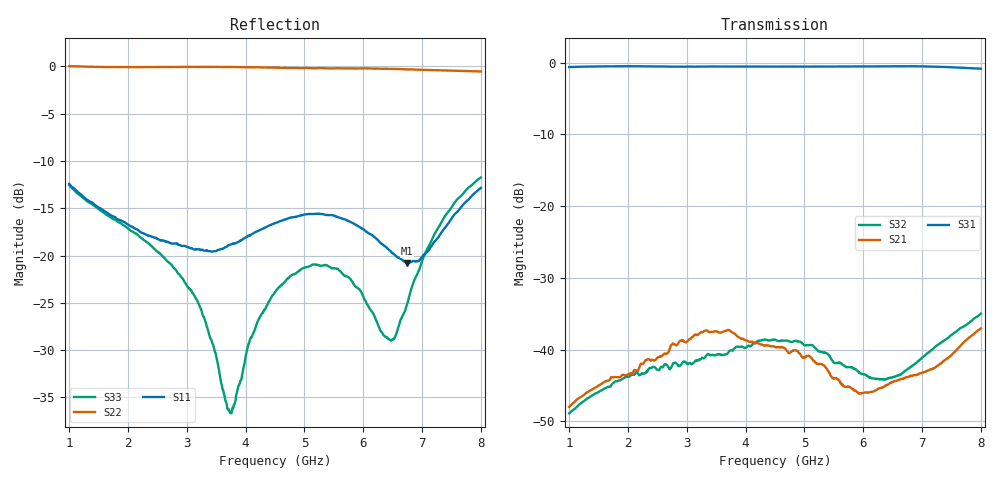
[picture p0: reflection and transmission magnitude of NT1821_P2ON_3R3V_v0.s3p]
! NT1821 PC-P2 ON state
! Port1:PC, Port2:P1, Port3:P2
! VDD=3.3V, VCTL=0V
# hz S ma R 50
! 3 Port Network Data from SP1.SP block
! freq  magS11  angS11  magS12  angS12  magS13  angS13
!  magS21  angS21
!  magS22  angS22  magS23  angS23
!  magS31  angS31  magS32  angS32
!  magS33  angS33
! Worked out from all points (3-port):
!   701 points, 1 GHz to 8 GHz, reference 50 ohm
!   strongest paths, dB at 1 GHz, 2.75 GHz, 4.5 GHz, 6.25 GHz, 8 GHz:
!     S31: -0.6, -0.6, -0.6, -0.5, -0.8
!     S21: -48.0, -39.3, -39.6, -45.4, -37.0
!     S32: -48.9, -42.2, -38.6, -44.1, -35.0
!   lowest |S11| = -20.8 dB at 6.75 GHz (marker M1), VSWR 1.20, Z = 47.4 - j8.51 ohm
!   |S11| at or under -10 dB: start of sweep to end of sweep
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1e9  0.2394 -78.5  0.004006 75.1  0.9327 2.1
     0.003986 75.0  1.002 -12.8  0.003596 72.7
     0.9321 2.0  0.0036 72.5  0.2358 -76.8
3.1e9  0.1086 -58.7  0.01234 70.8  0.9375 -25.1
       0.01228 70.6  0.9935 -36.5  0.007994 64.8
       0.9378 -25.3  0.00798 65.0  0.06349 -94.4
3.73e9  0.1139 -35.7  0.01366 50.3  0.9391 -31.2
        0.01362 49.9  0.9917 -42.9  0.009818 66.6
        0.9391 -31.6  0.009834 66.4  0.01483 -167.1
4.07e9  0.127 -28.3  0.01135 46.5  0.9405 -34.5
        0.01132 46.4  0.9893 -46.8  0.01054 63.0
        0.9403 -34.8  0.01056 62.7  0.03551 121.7
4.5e9  0.1482 -25.0  0.0105 45.2  0.9389 -38.9
       0.01046 45.2  0.9834 -52.6  0.01173 54.4
       0.9384 -39.4  0.01175 53.8  0.06405 104.5
5.55e9  0.1604 -35.5  0.006368 46.2  0.9402 -49.0
        0.006293 46.4  0.9765 -70.8  0.008006 47.9
        0.9397 -49.5  0.008055 46.8  0.0854 94.2
6.46e9  0.1058 -73.7  0.005883 95.0  0.9444 -58.5
        0.00588 95.3  0.97 -90.2  0.006346 84.1
        0.9445 -59.0  0.0064 83.8  0.03584 158.7
6.75e9  0.09103 -102.0  0.006459 103.4  0.9443 -61.6
        0.006439 103.3  0.9636 -96.1  0.007311 100.5
        0.9442 -62.4  0.007296 99.5  0.05552 -153.4
7.36e9  0.1367 -163.7  0.008297 126.7  0.9331 -68.9
        0.008301 126.3  0.9512 -106.8  0.01144 116.8
        0.933 -69.4  0.0114 116.8  0.1562 -130.6
8e9  0.2278 171.2  0.01408 136.1  0.9078 -76.0
     0.01406 136.2  0.9401 -114.6  0.01782 124.3
     0.9078 -76.4  0.01782 123.9  0.2586 -127.8
